|   stm32f0_448_wlcsp49 IBIS Model
[IBIS ver]   4.2
[File name]  stm32f0_448_wlcsp49.ibs
[File Rev]   1.0
[Date]   15-5-2013
[Source] Data Created at STMicroelectronics
[Notes]   File originated from ELDO simulations.
[Disclaimer]  This information is for modeling purpose only and is
   not guaranted. The information is subject to change without
   notice.
[Copyright] Copyright 2015 STMicroelectronics Inc.
[Component] stm32f0_448_wlcsp49
[Manufacturer] STMicroelectronics
[Package]
| variable   typ   min   max
R_pkg   0.0   NA   NA
L_pkg   0.0H   NA   NA
C_pkg   0.0F   NA   NA
[Pin] signal_name  model_name   R_pin   L_pin   C_pin
B7   VBAT   POWER   69.0E-3   4.2E-9   120.0E-15
D5   PC13   io8p_sudq_tc   61.9E-3   3.5E-9   84.0E-15
C7   PC14   io8p_sudq_tc   56.4E-3   2.9E-9   56.0E-15
C6   PC15   io8p_sudq_tc   52.4E-3   2.5E-9   36.0E-15
D7   PF0   io8p_sudq_ft   50.1E-3   2.3E-9   24.0E-15
D6   PF1   io8p_sudq_ft   49.3E-3   2.2E-9   20.0E-15
E7   NRST   ioreset_tc_v33   49.3E-3   2.2E-9   20.0E-15
E6   VSSA   GND   50.1E-3   2.3E-9   24.0E-15
F7   VDDA   POWER   52.4E-3   2.5E-9   36.0E-15
F6   PA0   io8p_sudq_ft   56.4E-3   2.9E-9   56.0E-15
G7   PA1   io8p_sudq_ft   61.9E-3   3.5E-9   84.0E-15
E5   PA2   io8p_sudq_ft   69.0E-3   4.2E-9   120.0E-15
E4   PA3   io8p_sudq_ft   69.0E-3   4.2E-9   120.0E-15
G6   PA4   io8p_sudq_ft   61.9E-3   3.5E-9   84.0E-15
F5   PA5   io8p_sudq_ft   56.4E-3   2.9E-9   56.0E-15
F4   PA6   io8p_sudq_ft   52.4E-3   2.5E-9   36.0E-15
F3   PA7   io8p_sudq_ft   50.1E-3   2.3E-9   24.0E-15
G5   PB0   io8p_sudq_ft   49.3E-3   2.2E-9   20.0E-15
G4   PB1   io8p_sudq_ft   49.3E-3   2.2E-9   20.0E-15
G3   PB2   io8p_sudq_ft   50.1E-3   2.3E-9   24.0E-15
E3   PB10   io8p_sudq_i2cin_lv_ft   52.4E-3   2.5E-9   36.0E-15
G2   PB11   io8p_sudq_i2cin_lv_ft   56.4E-3   2.9E-9   56.0E-15
D3   VSS   GND   61.9E-3   3.5E-9   84.0E-15
F2   VDD   POWER   69.0E-3   4.2E-9   120.0E-15
E2   PB12   io8p_sudq_ft   69.0E-3   4.2E-9   120.0E-15
G1   PB13   io8p_sudq_ft   61.9E-3   3.5E-9   84.0E-15
F1   PB14   io8p_sudq_ft   56.4E-3   2.9E-9   56.0E-15
E1   PB15   io8p_sudq_ft   52.4E-3   2.5E-9   36.0E-15
D1   PA8   io8p_sudq_ft   50.1E-3   2.3E-9   24.0E-15
D2   PA9   io8p_sudq_ft   49.3E-3   2.2E-9   20.0E-15
C2   PA10   io8p_sudq_ft   49.3E-3   2.2E-9   20.0E-15
C1   PA11   io8p_sudq_ft   50.1E-3   2.3E-9   24.0E-15
C3   PA12   io8p_sudq_ft   52.4E-3   2.5E-9   36.0E-15
B3   PA13   io8p_sudq_ft   56.4E-3   2.9E-9   56.0E-15
B1   VSS   GND   61.9E-3   3.5E-9   84.0E-15
B2   VDDIO2   POWER   69.0E-3   4.2E-9   120.0E-15
A1   PA14   io8p_sudq_ft   69.0E-3   4.2E-9   120.0E-15
A2   PA15   io8p_sudq_ft   61.9E-3   3.5E-9   84.0E-15
A3   PB3   io8p_sudq_ft   56.4E-3   2.9E-9   56.0E-15
A4   PB4   io8p_sudq_ft   52.4E-3   2.5E-9   36.0E-15
B4   PB5   io8p_sudq_ft   50.1E-3   2.3E-9   24.0E-15
C4   PB6   io8p_sudq_i2cin_lv_ft   49.3E-3   2.2E-9   20.0E-15
D4   PB7   io8p_sudq_i2cin_lv_ft   49.3E-3   2.2E-9   20.0E-15
A5   BOOT0   vpp_test_hv   50.1E-3   2.3E-9   24.0E-15
B5   PB8   io8p_sudq_i2cin_lv_ft   52.4E-3   2.5E-9   36.0E-15
C5   PB9   io8p_sudq_i2cin_lv_ft   56.4E-3   2.9E-9   56.0E-15
A6   VSS   GND   61.9E-3   3.5E-9   84.0E-15
A7   VDD   POWER   69.0E-3   4.2E-9   120.0E-15
[Model Selector] io8p_sudq_ft
io8p01_sudq_ft_pd_lv  "SPEED01 2P0V, PD=40kOhm"
io8p01_sudq_ft_pu_lv  "SPEED01 2P0V, PU=40kOhm"
io8p01_sudq_ft_lv  "SPEED01 2P0V"
io8p10_sudq_ft_pd_lv  "SPEED10 2P0V, PD=40kOhm"
io8p10_sudq_ft_pu_lv  "SPEED10 2P0V, PU=40kOhm"
io8p10_sudq_ft_lv  "SPEED10 2P0V"
io8p11_sudq_ft_pd_lv  "SPEED11 2P0V, PD=40kOhm"
io8p11_sudq_ft_pu_lv  "SPEED11 2P0V, PU=40kOhm"
io8p11_sudq_ft_lv  "SPEED11 2P0V"
io8p01_sudq_ft_pd  "SPEED01, PD=40kOhm"
io8p01_sudq_ft_pu  "SPEED01, PU=40kOhm"
io8p01_sudq_ft  "SPEED01"
io8p10_sudq_ft_pd  "SPEED10, PD=40kOhm"
io8p10_sudq_ft_pu  "SPEED10, PU=40kOhm"
io8p10_sudq_ft  "SPEED10"
io8p11_sudq_ft_pd  "SPEED11, PD=40kOhm"
io8p11_sudq_ft_pu  "SPEED11, PU=40kOhm"
io8p11_sudq_ft  "SPEED11"
[Model Selector] io8p_sudq_i2cin_lv_ft
io8p01_sudq_i2cin_lv_ft_pd_lv  "SPEED01 2P0V, PD=40kOhm"
io8p01_sudq_i2cin_lv_ft_pu_lv  "SPEED01 2P0V, PU=40kOhm"
io8p01_sudq_i2cin_lv_ft_lv  "SPEED01 2P0V"
io8p10_sudq_i2cin_lv_ft_pd_lv  "SPEED10 2P0V, PD=40kOhm"
io8p10_sudq_i2cin_lv_ft_pu_lv  "SPEED10 2P0V, PU=40kOhm"
io8p10_sudq_i2cin_lv_ft_lv  "SPEED10 2P0V"
io8p11_sudq_i2cin_lv_ft_pd_lv  "SPEED11 2P0V, PD=40kOhm"
io8p11_sudq_i2cin_lv_ft_pu_lv  "SPEED11 2P0V, PU=40kOhm"
io8p11_sudq_i2cin_lv_ft_lv  "SPEED11 2P0V"
io8p01_sudq_i2cin_lv_ft_pd  "SPEED01, PD=40kOhm"
io8p01_sudq_i2cin_lv_ft_pu  "SPEED01, PU=40kOhm"
io8p01_sudq_i2cin_lv_ft  "SPEED01"
io8p10_sudq_i2cin_lv_ft_pd  "SPEED10, PD=40kOhm"
io8p10_sudq_i2cin_lv_ft_pu  "SPEED10, PU=40kOhm"
io8p10_sudq_i2cin_lv_ft  "SPEED10"
io8p11_sudq_i2cin_lv_ft_pd  "SPEED11, PD=40kOhm"
io8p11_sudq_i2cin_lv_ft_pu  "SPEED11, PU=40kOhm"
io8p11_sudq_i2cin_lv_ft  "SPEED11"
[Model Selector] io8p_sudq_tc
io8p01_sudq_tc_pd_lv  "SPEED01 2P0V, PD=40kOhm"
io8p01_sudq_tc_pu_lv  "SPEED01 2P0V, PU=40kOhm"
io8p01_sudq_tc_lv  "SPEED01 2P0V"
io8p10_sudq_tc_pd_lv  "SPEED10 2P0V, PD=40kOhm"
io8p10_sudq_tc_pu_lv  "SPEED10 2P0V, PU=40kOhm"
io8p10_sudq_tc_lv  "SPEED10 2P0V"
io8p11_sudq_tc_pd_lv  "SPEED11 2P0V, PD=40kOhm"
io8p11_sudq_tc_pu_lv  "SPEED11 2P0V, PU=40kOhm"
io8p11_sudq_tc_lv  "SPEED11 2P0V"
io8p01_sudq_tc_pd  "SPEED01, PD=40kOhm"
io8p01_sudq_tc_pu  "SPEED01, PU=40kOhm"
io8p01_sudq_tc  "SPEED01"
io8p10_sudq_tc_pd  "SPEED10, PD=40kOhm"
io8p10_sudq_tc_pu  "SPEED10, PU=40kOhm"
io8p10_sudq_tc  "SPEED10"
io8p11_sudq_tc_pd  "SPEED11, PD=40kOhm"
io8p11_sudq_tc_pu  "SPEED11, PU=40kOhm"
io8p11_sudq_tc  "SPEED11"
[Model Selector] ioreset_tc_v33
ioreset_tc_v33_pu_lv  "IORESET 2V + PU=40kOhm"
ioreset_tc_v33_nopu_lv  "IORESET 2V"
ioreset_tc_v33_pu  "IORESET + PU=40kOhm"
ioreset_tc_v33_nopu  "IORESET"
[Model Selector] vpp_test_hv
vpp_test_hv_3p3  "Input Buffer"
vpp_test_hv_2p4  "Input Buffer 2P0V"
| Models and submodels in the file (60): io8p01_sudq_ft_pd_lv (I/O), io8p01_sudq_ft_pu_lv (I/O), io8p01_sudq_ft_lv (I/O), io8p10_sudq_ft_pd_lv (I/O), io8p10_sudq_ft_pu_lv (I/O), io8p10_sudq_ft_lv (I/O), io8p11_sudq_ft_pd_lv (I/O), io8p11_sudq_ft_pu_lv (I/O), io8p11_sudq_ft_lv (I/O), io8p01_sudq_ft_pd (I/O), io8p01_sudq_ft_pu (I/O), io8p01_sudq_ft (I/O), io8p10_sudq_ft_pd (I/O), io8p10_sudq_ft_pu (I/O), io8p10_sudq_ft (I/O), io8p11_sudq_ft_pd (I/O), io8p11_sudq_ft_pu (I/O), io8p11_sudq_ft (I/O), io8p01_sudq_i2cin_lv_ft_pd_lv (I/O), io8p01_sudq_i2cin_lv_ft_pu_lv (I/O), io8p01_sudq_i2cin_lv_ft_lv (I/O), io8p10_sudq_i2cin_lv_ft_pd_lv (I/O), io8p10_sudq_i2cin_lv_ft_pu_lv (I/O), io8p10_sudq_i2cin_lv_ft_lv (I/O), io8p11_sudq_i2cin_lv_ft_pd_lv (I/O), io8p11_sudq_i2cin_lv_ft_pu_lv (I/O), io8p11_sudq_i2cin_lv_ft_lv (I/O), io8p01_sudq_i2cin_lv_ft_pd (I/O), io8p01_sudq_i2cin_lv_ft_pu (I/O), io8p01_sudq_i2cin_lv_ft (I/O), io8p10_sudq_i2cin_lv_ft_pd (I/O), io8p10_sudq_i2cin_lv_ft_pu (I/O), io8p10_sudq_i2cin_lv_ft (I/O), io8p11_sudq_i2cin_lv_ft_pd (I/O), io8p11_sudq_i2cin_lv_ft_pu (I/O), io8p11_sudq_i2cin_lv_ft (I/O), io8p01_sudq_tc_pd_lv (I/O), io8p01_sudq_tc_pu_lv (I/O), io8p01_sudq_tc_lv (I/O), io8p10_sudq_tc_pd_lv (I/O), io8p10_sudq_tc_pu_lv (I/O), io8p10_sudq_tc_lv (I/O), io8p11_sudq_tc_pd_lv (I/O), io8p11_sudq_tc_pu_lv (I/O), io8p11_sudq_tc_lv (I/O), io8p01_sudq_tc_pd (I/O), io8p01_sudq_tc_pu (I/O), io8p01_sudq_tc (I/O), io8p10_sudq_tc_pd (I/O), io8p10_sudq_tc_pu (I/O), io8p10_sudq_tc (I/O), io8p11_sudq_tc_pd (I/O), io8p11_sudq_tc_pu (I/O), io8p11_sudq_tc (I/O), ioreset_tc_v33_pu_lv (I/O_open_drain), ioreset_tc_v33_nopu_lv (I/O_open_drain), ioreset_tc_v33_pu (I/O_open_drain), ioreset_tc_v33_nopu (I/O_open_drain), vpp_test_hv_2p4 (Input), vpp_test_hv_3p3 (Input)
